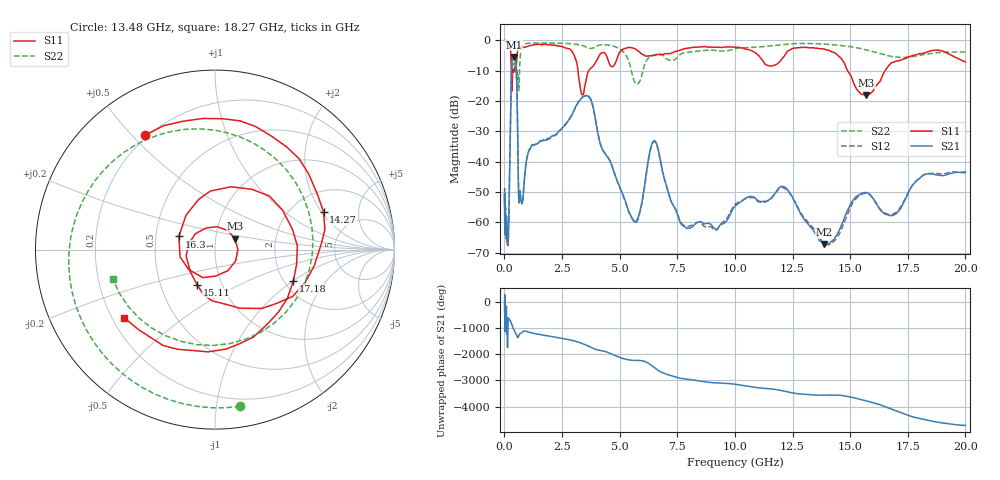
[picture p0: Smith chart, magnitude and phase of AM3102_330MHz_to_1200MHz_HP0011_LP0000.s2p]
! Date/Time: Tue, Sep 11, 2018 5:11 PM
! Network Analyzer: Agilent Technologies E8362B Rev: A.07.50.63
! Sweep from 0.010 to 20.000 GHz, 1601 Points, Sweep Type: LOG
! Power Supply: 4.949 V, 0.001 A
# Hz S DB R 50
!freq MagS11 AngS11 MagS21 AngS21 MagS12 AngS12 MagS22 AngS22
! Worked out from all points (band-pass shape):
!   1601 points, 10 MHz to 20 GHz, reference 50 ohm
!   highest |S21| = -5.40 dB at 402.8 MHz (marker M1); lowest = -67.2 dB at 13.87 GHz (marker M2)
!   |S21| within 3 dB of the highest: 320.1 MHz to 512.3 MHz (192.3 MHz wide, 46.2 % of centre)
!   lowest |S11| = -18.0 dB at 15.7 GHz (marker M3), VSWR 1.29, Z = 62 + j7.65 ohm
!   |S11| at or under -10 dB: 298.9 MHz to 358 MHz (59.14 MHz wide, 18 % of centre); 3.191 GHz to 3.655 GHz (463.2 MHz wide, 13.5 % of centre); 14.89 GHz to 16.51 GHz (1.62 GHz wide, 10.3 % of centre)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
!   |S22| runs from -16.5 to -0.2 dB; largest |S21 - S12| = 0.0068
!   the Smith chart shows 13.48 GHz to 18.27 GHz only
!   S11 on the Smith chart (normalised r, x): 13.48 GHz: 0.19, +0.55; 14.27 GHz: 2.95, +2.10; 15.11 GHz: 0.76, -0.31; 16.3 GHz: 0.66, +0.10; 17.18 GHz: 2.24, -1.00; 18.27 GHz: 0.25, -0.32
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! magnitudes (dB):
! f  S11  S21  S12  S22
! 10 MHz  0.0  -50.5  -49.3  -0.2
! 35.55 MHz  0.0  -61.7  -59.6  -0.3
! 126.4 MHz  -0.4  -62.7  -65.6  -0.7
! 174.6 MHz  -0.9  -63.1  -65.4  -1.1
! 402.8 MHz  -10.4  -5.4  -5.5  -7.9
! 447.2 MHz  -9.0  -5.8  -5.9  -7.4
! 530.6 MHz  -7.1  -11.5  -11.5  -12.5
! 635.6 MHz  -2.3  -53.4  -53.5  -15.9
! 1.59 GHz  -1.4  -33.1  -33.1  -0.8
! 3.634 GHz  -10.3  -18.4  -18.2  -2.4
! 5.652 GHz  -2.7  -59.7  -59.9  -13.7
! 6.518 GHz  -4.9  -33.0  -33.3  -4.7
! 7.845 GHz  -2.7  -61.5  -61.1  -4.0
! 13.48 GHz  -2.5  -63.7  -62.7  -1.1
! 13.87 GHz  -2.8  -67.2  -67.1  -1.2
! 14.27 GHz  -3.9  -65.7  -66.4  -1.4
! 15.11 GHz  -13.2  -52.9  -53.5  -2.2
! 15.7 GHz  -18.0  -50.2  -50.4  -3.1
! 16.3 GHz  -13.4  -55.9  -55.6  -4.3
! 17.18 GHz  -6.6  -55.5  -55.0  -5.6
! 18.27 GHz  -4.0  -44.1  -44.1  -4.5
! 20 GHz  -7.1  -43.3  -43.7  -3.8
